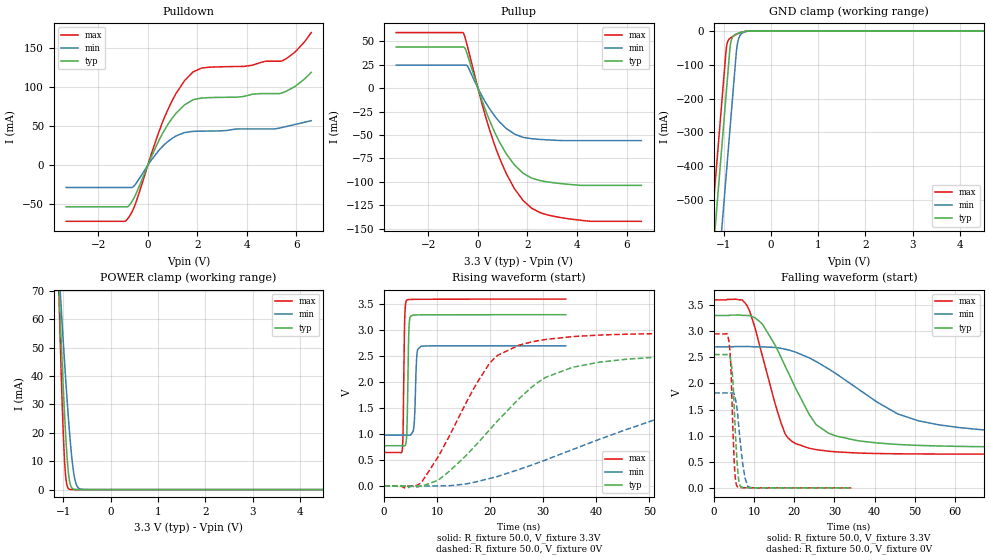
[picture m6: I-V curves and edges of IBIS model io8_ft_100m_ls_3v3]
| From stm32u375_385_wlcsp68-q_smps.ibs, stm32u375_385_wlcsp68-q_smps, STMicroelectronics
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[Model]   io8_ft_100m_ls_3v3
Model_type I/O
Polarity   Non-Inverting
Enable   Active-Low
| CAP_THRESHOLD on pad IOFT is "UDTCAPC" :
| Rising=30.0% of vddiom   Falling=70.0% of vddiom
| C_comp min and max val. don't necessarily correlate with the min and max pvt
| but are the smallest and greatest pad capacitance found.
| var   typ   min   max
C_comp   3.79549pF  3.74407pF  3.79817pF
|C_comp_pullup   2.32751pF  2.17276pF  2.40170pF
|C_comp_pulldown   1.46798pF  1.57131pF  1.39646pF
Vinl = 1.35V
Vinh = 1.8V
Vmeas = 1.65V   | Reference voltage for timing measurements
Cref  = 50.0pF   | Timing specification test load capacitance value
Rref  = 1.0MOhm   | Timing specification test load resistance value
Vref  = 1.815V   | Timing specification test load voltage
[Model Spec]
| TIME_THRESHOLD on pin ZIV11 is "CMOS" :
| Rising=50.0% of vdd   Falling=50.0% of vdd
Vinl 1.27950V 1.06950V 1.36550V
Vinh 1.78950V 1.51350V 1.89450V
| variable   typ   min   max
[Temperature Range] 25.0 130.0 -40.0
| variable   typ   min   max
[Voltage Range] 3.3V 2.7V 3.6V
| variable   typ   min   max
[POWER Clamp Reference] 3.3V 2.7V 3.6V
| variable   typ   min   max
[GND Clamp Reference] 0V 0V 0V
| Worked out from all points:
|   slope of the pulldown table from 0 to 0.495 V, typ, clamps not added: 14.3 ohm
|   slope of the pullup table from 0 to 0.495 V, typ, clamps not added: 13.8 ohm
|   GND clamp passes 1 mA (typ) near -0.50 V on its own axis
|   POWER clamp passes 1 mA (typ) near -0.83 V on its own axis
|   rising waveform, R_fixture 50.0, V_fixture 3.3V: 20-80 % time 256ps typ, 338ps min, 238ps max; typ from 0.776 V to 3.3 V
|   falling waveform, R_fixture 50.0, V_fixture 3.3V: 20-80 % time 10.1ns typ, 22.5ns min, 6.33ns max; typ from 3.3 V to 0.776 V
|   rising waveform, R_fixture 50.0, V_fixture 0V: 20-80 % time 15ns typ, 30.8ns min, 9.54ns max; typ from 0 V to 2.55 V
|   falling waveform, R_fixture 50.0, V_fixture 0V: 20-80 % time 1.03ns typ, 1.53ns min, 819ps max; typ from 2.55 V to 0 V
[POWER Clamp]
-3.3V     1.126A     769.5mA    1.647A
-1.1V     75.38mA    79.63mA    73.18mA
-1.09V    71.2mA     76.8mA     67.14mA
-1.08V    67.05mA    73.98mA    61.2mA
-1.06V    58.89mA    68.38mA    49.67mA
-1.01V    39.47mA    54.71mA    24.03mA
-970mV    25.49mA    44.18mA    9.257mA
-930mV    13.81mA    34.16mA    2.168mA
-870mV    3.251mA    20.56mA    140.6uA
-760mV    67.19uA    3.98mA     739.8nA
-630mV    518.7nA    149.1uA    1.803nA
6.6V      0A         0A         0A
[GND Clamp]
-3.3V     -4.191A    -4.432A    -4.059A
-1.25V    -706mA     -946.8mA   -573.6mA
-950mV    -196mA     -436.8mA   -63.63mA
-940mV    -179mA     -419.8mA   -50.26mA
-910mV    -128mA     -368.8mA   -31.05mA
-850mV    -37.37mA   -266.8mA   -20.53mA
-810mV    -18.79mA   -198.8mA   -16.88mA
-720mV    -8.735mA   -51.28mA   -10.12mA
-680mV    -6.635mA   -22.61mA   -7.598mA
-630mV    -4.51mA    -9.474mA   -4.925mA
-400mV    -114.4uA   -369.6uA   -46.93uA
6.6V      2.22nA     299.7nA    1.002nA
| variable   typ   min   max
[Pullup Reference] 3.3V 2.7V 3.6V
| variable   typ   min   max
[Pulldown Reference] 0V 0V 0V
[Pullup]
-3.3V     43.8mA     24.59mA    59.28mA
-590mV    43.8mA     24.59mA    58.78mA
-520mV    42.4mA     24.59mA    54mA
-410mV    34.51mA    22.84mA    43.15mA
310mV     -23.64mA   -15.21mA   -30.46mA
880mV     -58mA      -36.24mA   -75.16mA
1.48V     -82.17mA   -49.14mA   -107.6mA
1.83V     -90.96mA   -52.61mA   -120.1mA
2.17V     -96.08mA   -54mA      -128.2mA
2.85V     -100.3mA   -55.28mA   -135.6mA
3.88V     -103.2mA   -56.04mA   -140.2mA
6.6V      -103.8mA   -56.04mA   -142.1mA
[Pulldown]
-3.3V     -53.27mA   -28.52mA   -71.84mA
-840mV    -53.27mA   -28.52mA   -69.65mA
-500mV    -38.18mA   -24.47mA   -49.51mA
460mV     32.61mA    19.53mA    43.99mA
800mV     51.7mA     30.09mA    70.55mA
1.14V     66.56mA    37.47mA    92mA
1.48V     77.24mA    41.82mA    108.3mA
1.83V     83.91mA    43.43mA    119.6mA
2.17V     86.16mA    43.73mA    124.5mA
5.39V     92.36mA    48.12mA    133.3mA
5.93V     100.6mA    52.1mA     144.5mA
6.6V      119.1mA    57.05mA    170mA
[Ramp]
dV/dt_r 1.53142V/14.92484ns 1.09007V/30.62057ns 1.76896V/9.52099ns
dV/dt_f 1.51461V/9.92031ns 1.03179V/22.12768ns 1.77292V/6.31505ns
R_load = 50.0
| Removed startup time: 0s 0s 0s  .
| Removed end time: 34.25ns.
[Rising Waveform]
R_fixture   = 50.0
V_fixture   = 3.3V
V_fixture_min = 2.7V
V_fixture_max = 3.6V
0s        775.7mV    980.2mV    645.1mV
3.45ns    775.6mV    980.2mV    694.8mV
3.9ns     774.7mV    980.2mV    3.18V
4.3ns     997.8mV    980.2mV    3.58V
4.65ns    2.86V      979.8mV    3.592V
5ns       3.269V     978.1mV    3.594V
5.7ns     3.294V     1.209V     3.595V
6.25ns    3.296V     2.57V      3.596V
7ns       3.297V     2.693V     3.597V
34.25ns   3.3V       2.7V       3.6V
| Removed startup time: 0s 0s 0s  .
| Removed end time: 249.25ns.
[Falling Waveform]
R_fixture   = 50.0
V_fixture   = 3.3V
V_fixture_min = 2.7V
V_fixture_max = 3.6V
0s        3.3V       2.7V       3.6V
7.75ns    3.301V     2.706V     3.539V
8.9ns     3.299V     2.704V     3.375V
11.7ns    3.162V     2.7V       2.623V
17.8ns    2.317V     2.654V     1.025V
25.45ns   1.208V     2.419V     732.4mV
30.55ns   989.8mV    2.178V     688.7mV
45.85ns   830.4mV    1.412V     652mV
66.15ns   788.8mV    1.117V     646.1mV
249.3ns   775.7mV    980.3mV    645.1mV
| Removed startup time: 0s 0s 0s  .
| Removed end time: 249.25ns.
[Rising Waveform]
R_fixture   = 50.0
V_fixture   = 0V
V_fixture_min = 0V
V_fixture_max = 0V
0s        11.22nV    82.64nV    22.9nV
6.35ns    -973uV     -18.52mV   19.47mV
10.2ns    108.9mV    -3.722uV   558.9mV
20.35ns   1.134V     155.6mV    2.415V
25.45ns   1.682V     317.5mV    2.713V
30.55ns   2.097V     504.9mV    2.824V
40.55ns   2.384V     898mV      2.907V
55.95ns   2.502V     1.419V     2.939V
76.3ns    2.541V     1.684V     2.947V
249.3ns   2.552V     1.817V     2.948V
| Removed startup time: 0s 0s 0s  .
| Removed end time: 34.2ns.
[Falling Waveform]
R_fixture   = 50.0
V_fixture   = 0V
V_fixture_min = 0V
V_fixture_max = 0V
0s        2.552V     1.817V     2.948V
3.65ns    2.554V     1.817V     2.824V
4.15ns    2.438V     1.817V     2.368V
4.65ns    2.098V     1.818V     1.219V
5.1ns     1.401V     1.771V     397.4mV
5.8ns     425mV      1.462V     23.74mV
6.5ns     36.43mV    896.4mV    5.183mV
7.7ns     3.292mV    193.8mV    3.035mV
8.4ns     2.345mV    29.86mV    2.99mV
34.2ns    161.3uV    246.3uV    125uV
